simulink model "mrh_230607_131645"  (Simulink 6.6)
settings: Solver=VariableStepDiscrete  StartTime=0.0  StopTime=0.0  RelTol=1e-3
libraries: ltpda_library x2

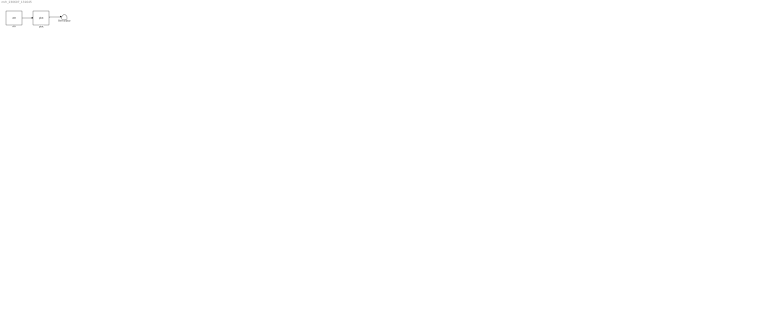
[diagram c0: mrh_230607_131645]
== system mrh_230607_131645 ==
  note: .
  AO : ltpda_library/AO  Tag=input  SystemSampleTime=-1
  Terminator : Terminator
  plot : ltpda_library/plot  SystemSampleTime=-1
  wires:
  AO/1 -> plot/1
  plot/1 -> Terminator/1
